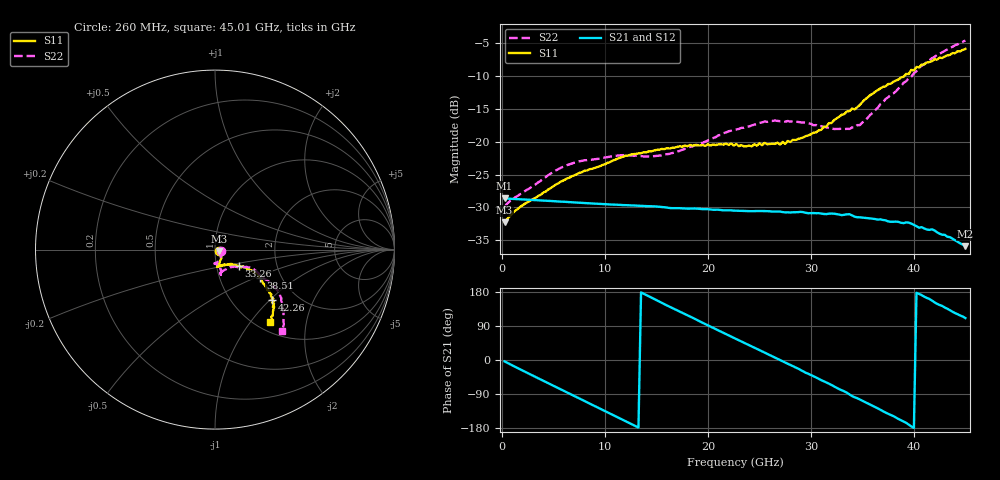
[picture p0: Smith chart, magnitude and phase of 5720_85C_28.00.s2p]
! Device:  ADRF5720
! Description: 0.5dB LSB GaAs MMIC 6-bit Digital Attenuator
! Frequency:  0.000009 -  40 GHz
! Ports:
!	RF1	= Port 1
!	RF2	= Port 2
! Vdd:  3.3 Volt
! Vss:  -3.3 Volt
! Control:  0/3.3 Volt
! State:  28.00 dB attenuation
! Data:  The device was measured using G-S-G Probes on a matrix board.
!  Data was collected using an calibrated 4 port network analyzer.
!  The reference plane for this measurement is at the launchers.
! Note:  Analog Devices supplies this data as a sample of measured data
!  for this product.  Your particular data for this product may vary.
!  Data was taken at 85 degrees C.
!  Analog Devices reserves the right to change this data at anytime.
# GHZ S DB R 45.0
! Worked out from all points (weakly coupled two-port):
!   180 points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, 260 MHz to 45.01 GHz, reference 45 ohm
!   highest |S21| = -28.63 dB at 260 MHz (marker M1); lowest = -35.9 dB at 45.01 GHz (marker M2)
!   lowest |S11| = -32.3 dB at 260 MHz (marker M3), VSWR 1.05, Z = 47.1 - j0.734 ohm
!   |S11| at or under -10 dB: start of sweep to 39.08 GHz
!   |S22| runs from -29.9 to -4.6 dB; largest |S21 - S12| = 0.00024
!   S11 on the Smith chart (normalised r, x): 260 MHz: 1.05, -0.02; 33.26 GHz: 1.28, -0.24; 38.51 GHz: 1.56, -0.54; 42.26 GHz: 1.51, -1.02; 45.01 GHz: 1.15, -1.25
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0.26  -32.27 -18.6  -28.63 -3.8  -28.63 -3.7  -29.91 -15.9
1.76  -29.93 -4.9  -28.76 -24.4  -28.75 -24.4  -27.99 -19.2
5.01  -26.75 -38.3  -29.04 -68.1  -29.03 -68.0  -24.58 -63.3
7.76  -24.65 -53.8  -29.30 -104.7  -29.28 -104.7  -22.91 -80.5
12.01  -22.13 -71.0  -29.65 -161.3  -29.64 -161.2  -22.03 -92.0
15.26  -21.22 -78.9  -29.89 154.4  -29.88 154.6  -22.11 -87.3
18.26  -20.49 -82.2  -30.17 114.9  -30.16 115.1  -20.79 -78.6
22.76  -20.34 -78.0  -30.49 55.2  -30.47 55.4  -18.12 -74.3
24.26  -20.71 -74.7  -30.57 36.0  -30.55 36.2  -17.52 -75.4
25.51  -20.17 -69.5  -30.55 19.5  -30.54 19.7  -16.93 -77.2
27.51  -20.33 -61.0  -30.75 -6.8  -30.73 -6.5  -16.95 -77.3
27.76  -19.88 -57.7  -30.74 -9.9  -30.72 -9.6  -16.84 -78.3
30.26  -18.63 -46.0  -30.85 -42.8  -30.82 -42.6  -17.50 -77.1
33.26  -15.78 -34.5  -31.10 -82.9  -31.09 -82.6  -18.06 -58.4
34.76  -14.39 -31.5  -31.50 -104.4  -31.48 -104.0  -17.47 -45.6
35.76  -12.91 -30.0  -31.67 -117.7  -31.65 -117.3  -15.92 -37.7
37.76  -11.18 -29.6  -32.18 -145.0  -32.17 -144.8  -12.86 -27.5
38.51  -10.53 -31.9  -32.20 -155.7  -32.19 -155.3  -11.91 -27.3
40.26  -8.61 -37.1  -32.85 177.3  -32.80 177.7  -9.26 -30.6
42.26  -7.51 -41.3  -33.79 148.1  -33.81 148.4  -6.77 -36.3
43.51  -6.78 -44.0  -34.52 131.2  -34.49 131.7  -5.68 -42.7
45.01  -5.88 -53.0  -35.89 110.5  -35.83 111.1  -4.59 -50.4
